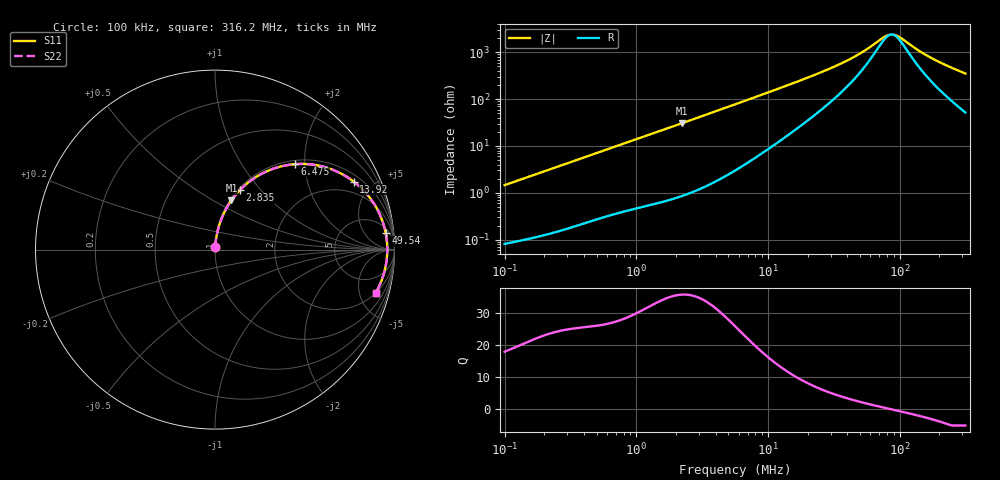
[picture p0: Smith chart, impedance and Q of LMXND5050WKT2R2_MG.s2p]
! LMXND5050WKT2R2_MG  S-PARAMETER MODEL  ( General Type )
! Model Generated by TAIYO YUDEN Corporation (http://www.ty-top.com)
! Version 1.0
! TAIYO YUDEN Control No. 191023NI43SB-FBB
! Copyright(c) 2019 TAIYO YUDEN CO.,LTD. All Rights Reserved.
! Product Description (link to TY-COMPAS)
! https://ds.yuden.co.jp/TYCOMPAS/or/detail?pn=LMXND5050WKT2R2NMG&u=M
! Products Name : Inductors
! Characteristics :
!  Inductance : 2.2 uH , SRF(min) : 57 MHz , DC Resistance(max) : 0.042 Ohm
!  Rated Current : Saturation :2900 mA , Temp Rise : 2900 mA
!  Case Size : 4.9 x 4.9 / 0.193 x 0.193 [mm/inch] , Thickness : 2 / 0.079 [mm/inch]
!  (Conditions: Temperature = 25 degC , DC Bias Current/Voltage = 0A / 0V)
! External Node Assignments :
!  1  o---GGG---o  2
! GND o---------o GND
! Frequency Range : 0.1MHz  -  316.199832MHz  [ 402 STEP ]
# MHz S RI R 50
! Freq[MHz].  S11 Real  S11 Imag  S21 Real  S21 Imag  S12 Real  S12 Imag  S22 Real  S22 Imag
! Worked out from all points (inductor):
!   401 points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, 100 kHz to 316.2 MHz, reference 50 ohm
!   read as one part in series: L = 2.31 uH near 104.1 kHz
!   highest Q = 35.7 at 2.226 MHz (marker M1), where L = 2.19 uH
!   self-resonance near 87.19 MHz
!   S11 on the Smith chart (normalised r, x): 100 kHz: 1.00, +0.03; 2.835 MHz: 1.02, +0.78; 6.475 MHz: 1.08, +1.78; 13.92 MHz: 1.33, +3.88; 49.54 MHz: 8, +17; 316.2 MHz: 2.03, -6.97
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0.1  0.00102 0.0146  0.999 -0.0146  0.999 -0.0146  0.00102 0.0146
0.385695  0.00511 0.0543  0.9949 -0.0543  0.9949 -0.0543  0.00511 0.0543
0.7966  0.016 0.1088  0.984 -0.1088  0.984 -0.1088  0.016 0.1088
1.487603  0.0457 0.1944  0.9543 -0.1944  0.9543 -0.1944  0.0457 0.1944
2.225795  0.0919 0.2752  0.9081 -0.2752  0.9081 -0.2752  0.0919 0.2752
2.83455  0.1384 0.3314  0.8616 -0.3314  0.8616 -0.3314  0.1384 0.3314
3.992385  0.2379 0.4102  0.7621 -0.4102  0.7621 -0.4102  0.2379 0.4102
5.623165  0.3784 0.4661  0.6216 -0.4661  0.6216 -0.4661  0.3784 0.4661
6.474856  0.4447 0.476  0.5553 -0.476  0.5553 -0.476  0.4447 0.476
9.119657  0.6077 0.4608  0.3923 -0.4608  0.3923 -0.4608  0.6077 0.4608
13.9228  0.7729 0.379  0.2271 -0.379  0.2271 -0.379  0.7729 0.379
21.68824  0.8787 0.2665  0.1213 -0.2665  0.1213 -0.2665  0.8787 0.2665
34.47245  0.9323 0.16  0.0677 -0.16  0.0677 -0.16  0.9323 0.16
49.54165  0.9512 0.0912  0.0488 -0.0912  0.0488 -0.0912  0.9512 0.0912
75.63424  0.9595 0.022  0.0405 -0.022  0.0405 -0.022  0.9595 0.022
83.65039  0.9599 0.0064  0.0401 -0.0064  0.0401 -0.0064  0.9599 0.0064
88.86233  0.96 -0.00294  0.04 0.00294  0.04 0.00294  0.96 -0.00294
96.32018  0.9597 -0.0154  0.0403 0.0154  0.0403 0.0154  0.9597 -0.0154
138.4253  0.9543 -0.0735  0.0457 0.0735  0.0457 0.0735  0.9543 -0.0735
169.3225  0.9475 -0.1088  0.0525 0.1088  0.0525 0.1088  0.9475 -0.1088
233.7293  0.928 -0.1723  0.072 0.1723  0.072 0.1723  0.928 -0.1723
316.1998  0.8949 -0.2413  0.1051 0.2413  0.1051 0.2413  0.8949 -0.2413
